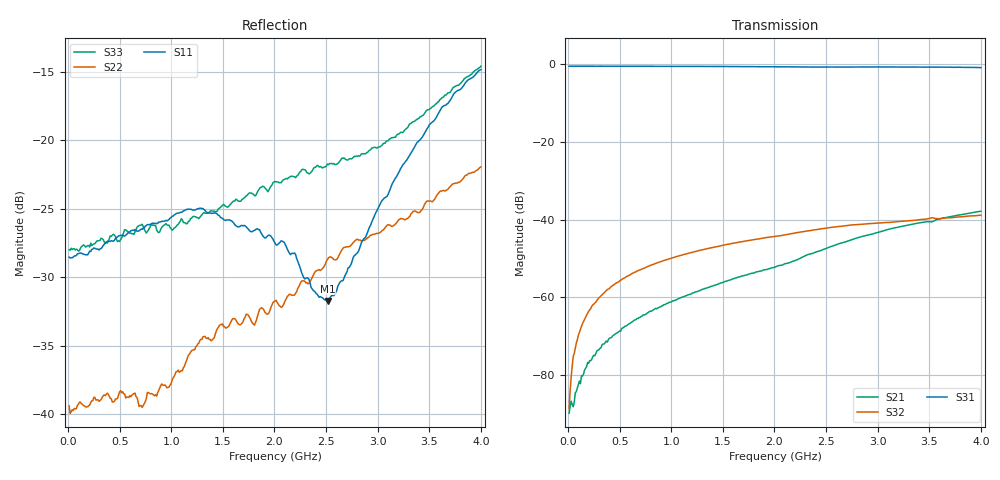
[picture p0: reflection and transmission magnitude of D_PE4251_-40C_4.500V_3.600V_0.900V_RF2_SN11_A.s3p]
! Device ID: PE4251_SoldCshunt_081809
! Dir: c:\Test Bench Repositories\Bench_Software_CVI_Version_8\trunk\PSC 4Port_VNA Bench\datalog\4250\TEST\PE4251_SoldCshunt_081809\-40C\4p500000\RF2
! Serial: 11
! Insertion: A
! Temp: -40C
! VDD: 4.500
! Control_Hi: 80.000
! Control_Lo: 20.000
! Logic State: RF2
! Port 1: RFC
! Port 2: RF1
! Port 3: RF2
! V1 = 0.90
! V2 = 0.90
! V3 = 0.90
! IDD: 5.419350e-05
! FILE NAME
! DATE 08/18/09  20:10
! CORRECTED  DATA
#  Hz  S  RI  R  50.00
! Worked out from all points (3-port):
!   401 points, 10 MHz to 4 GHz, reference 50 ohm
!   strongest paths, dB at 10 MHz, 1.008 GHz, 2.005 GHz, 3.002 GHz, 4 GHz:
!     S31: -0.5, -0.5, -0.6, -0.7, -0.8
!     S32: -88.7, -49.9, -44.3, -40.8, -38.8
!     S21: -89.8, -61.0, -52.2, -43.3, -37.8
!   lowest |S11| = -31.7 dB at 2.514 GHz (marker M1), VSWR 1.05, Z = 50.5 - j2.56 ohm
!   |S11| at or under -10 dB: start of sweep to end of sweep
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1e7  0.0375 -0.00059  8.72e-05 2.28e-06  0.9454 -0.00374
     2.42e-05 -2.13e-05  0.0107 -0.000795  6.76e-05 -6.42e-06
     0.9452 -0.00463  -2.65e-05 -2.56e-05  0.0399 0.000512
9.9775e7  0.0385 0.00189  1.03e-05 -7.01e-05  0.9445 -0.0364
          7.76e-06 -7.48e-05  0.0109 0.00025  3.56e-05 0.000325
          0.9456 -0.0359  2.78e-05 0.000325  0.0394 -0.0001
1.79575e8  0.0381 0.00335  -1.84e-05 -0.000131  0.9424 -0.0633
           -7.14e-06 -0.000128  0.0106 0.00117  3.84e-05 0.00059
           0.9432 -0.063  4.15e-05 0.000592  0.041 0.000705
4.888e8  0.0444 0.00555  -0.000185 -0.000324  0.9277 -0.1684
         -0.000175 -0.000313  0.0113 0.00291  0.000146 0.0016
         0.9276 -0.1681  0.000152 0.00158  0.0429 -0.00246
7.18225e8  0.0473 0.00233  -0.000393 -0.000423  0.9104 -0.2442
           -0.000395 -0.00042  0.00992 0.00369  0.000278 0.00231
           0.911 -0.2441  0.00027 0.00232  0.0491 -0.00532
1.2868e9  0.0559 -0.00855  -0.00112 -0.000549  0.8371 -0.4224
          -0.00111 -0.000548  0.0169 0.00811  0.000706 0.00399
          0.8398 -0.4223  0.000711 0.00401  0.0523 -0.00858
2.005e9  0.0381 -0.0182  -0.00234 -0.000758  0.7014 -0.6081
         -0.00233 -0.00075  0.0164 0.02  0.00128 0.00596
         0.7041 -0.6075  0.00127 0.00597  0.0649 -0.0283
2.513725e9  0.00554 -0.0253  -0.00414 -0.00125  0.589 -0.7086
            -0.00415 -0.00126  0.0182 0.0319  0.00179 0.00763
            0.591 -0.7088  0.00179 0.00763  0.053 -0.0625
3.371575e9  -0.0894 -0.0372  -0.00895 0.000218  0.3582 -0.8494
            -0.00895 0.000219  -0.000646 0.055  0.00269 0.00948
            0.3603 -0.8501  0.00268 0.0095  -0.0188 -0.1173
4e9  -0.1801 -0.0222  -0.0127 0.00261  0.1359 -0.8964
     -0.0126 0.00258  -0.0295 0.0744  0.00288 0.011
     0.1387 -0.8965  0.0029 0.0111  -0.1283 -0.1357
